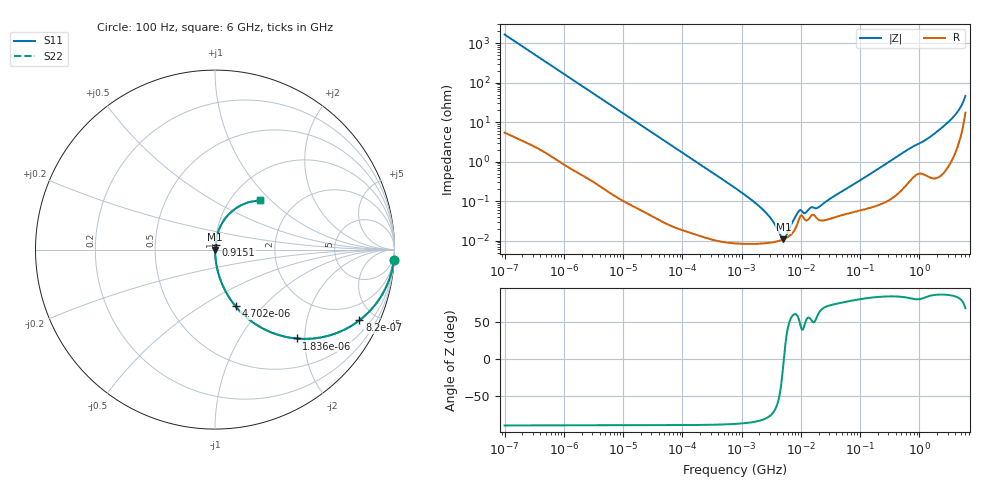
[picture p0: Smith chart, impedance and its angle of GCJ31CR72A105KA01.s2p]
!Murata Part Number: GCJ31CR72A105KA01
!These Parameters are Measured in Series Mode Connection
!Data Generated on Mar 13, 2026
!  o--ll--o
!Port1  Port2
!  o------o
!Operation Temp=25[degC], DC Bias Voltage=0[V]
!Freq. Start=100[Hz] Stop=6[GHz] 401[Steps]
# Hz S RI R 50
!Freq.(Hz) S11(Real) S11(Imag) S21(Real) S21(Imag) S12(Real) S12(Imag) S22(Real) S22(Imag)
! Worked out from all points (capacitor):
!   401 points, 100 Hz to 6 GHz, reference 50 ohm
!   read as one part in series: C = 957 nF near 109 Hz
!   lowest |Z| = 10.9 mohm at 5.079 MHz (marker M1)
!   series resonance near 5.178 MHz, so ESL is about 990 pH
!   S11 on the Smith chart (normalised r, x): 100 Hz: 1, -33; 820 Hz: 1.02, -4.08; 1.836 kHz: 1.01, -1.83; 4.702 kHz: 1.00, -0.72; 915.1 MHz: 1.01, +0.05; 6 GHz: 1.35, +0.86
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100  0.9962 -0.0599  0.0038 0.0599  0.0038 0.0599  0.9962 -0.0599
366  0.953 -0.2092  0.047 0.2092  0.047 0.2092  0.953 -0.2092
820  0.8048 -0.3938  0.1952 0.3938  0.1952 0.3938  0.8048 -0.3938
1836  0.4548 -0.4953  0.5452 0.4953  0.5452 0.4953  0.4548 -0.4953
2008  0.4112 -0.4893  0.5888 0.4893  0.5888 0.4893  0.4112 -0.4893
4702  0.1149 -0.316  0.8851 0.316  0.8851 0.316  0.1149 -0.316
12592  0.0184 -0.1314  0.9816 0.1314  0.9816 0.1314  0.0184 -0.1314
40335  0.00209 -0.0419  0.9979 0.0419  0.9979 0.0419  0.00209 -0.0419
774597  8.99e-05 -0.00216  0.9999 0.00216  0.9999 0.00216  8.99e-05 -0.00216
2481164  8.6e-05 -0.000537  0.9999 0.000537  0.9999 0.000537  8.6e-05 -0.000537
5079039  0.000108 -1.32e-05  0.9999 1.32e-05  0.9999 1.32e-05  0.000108 -1.32e-05
5554849  0.000115 4.9e-05  0.9999 -4.9e-05  0.9999 -4.9e-05  0.000115 4.9e-05
9090158  0.00031 0.000443  0.9997 -0.000443  0.9997 -0.000443  0.00031 0.000443
1.189169e7  0.000331 0.000376  0.9997 -0.000376  0.9997 -0.000376  0.000331 0.000376
1.555665e7  0.000451 0.000542  0.9995 -0.000542  0.9995 -0.000542  0.000451 0.000542
2.035112e7  0.000336 0.000632  0.9997 -0.000632  0.9997 -0.000632  0.000336 0.000632
3.124326e8  0.00117 0.00996  0.9988 -0.00996  0.9988 -0.00996  0.00117 0.00996
9.150511e8  0.00542 0.0265  0.9946 -0.0265  0.9946 -0.0265  0.00542 0.0265
1.497423e9  0.00569 0.0411  0.9943 -0.0411  0.9943 -0.0411  0.00569 0.0411
3.065283e9  0.0168 0.0971  0.9832 -0.0971  0.9832 -0.0971  0.0168 0.0971
4.586474e9  0.061 0.1786  0.939 -0.1786  0.939 -0.1786  0.061 0.1786
6e9  0.2491 0.2748  0.7509 -0.2748  0.7509 -0.2748  0.2491 0.2748
